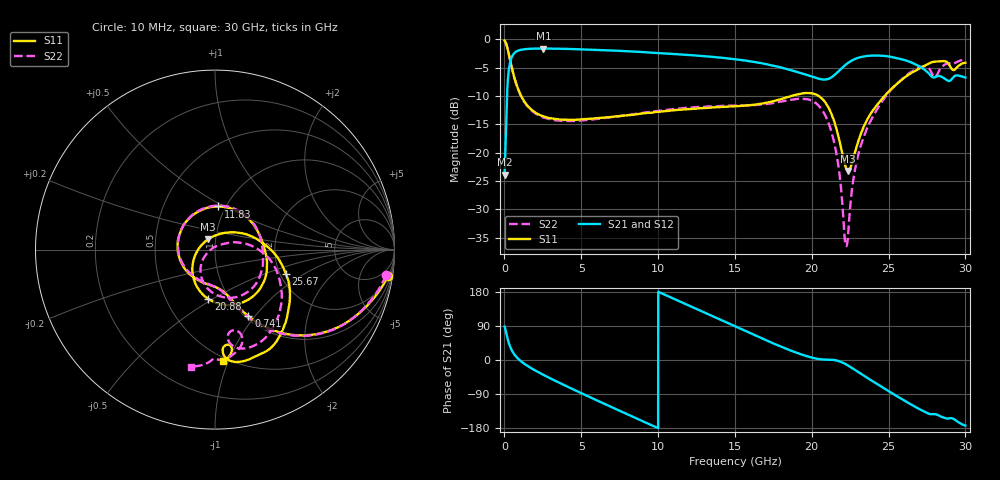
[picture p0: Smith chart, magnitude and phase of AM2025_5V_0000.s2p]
!Keysight Technologies,N5245B,MY58422270,A.16.20.02
!Date: Tuesday, July 14, 2026 00:49:01
!Correction: S11(C  2-Port  )
!S21(C  2-Port  )
!S12(C  2-Port  )
!S22(C  2-Port  )
!S2P File: Measurements: S11, S21, S12, S22:
# Hz S  dB  R 50
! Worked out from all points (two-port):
!   3201 points, 10 MHz to 30 GHz, reference 50 ohm
!   highest |S21| = -1.65 dB at 2.531 GHz (marker M1); lowest = -23.9 dB at 10 MHz (marker M2)
!   |S21| within 3 dB of the highest: 327.9 MHz to 17.47 GHz (17.14 GHz wide, 193 % of centre); 22.14 GHz to 26.91 GHz (4.765 GHz wide, 19.4 % of centre)
!   lowest |S11| = -23.2 dB at 22.37 GHz (marker M3), VSWR 1.15, Z = 46 + j5.25 ohm
!   |S11| at or under -10 dB: 1.086 GHz to 18.69 GHz (17.6 GHz wide, 178 % of centre); 20.45 GHz to 24.74 GHz (4.295 GHz wide, 19 % of centre)
!   |S22| runs from -36.5 to -0.3 dB; largest |S21 - S12| = 0.014
!   S11 on the Smith chart (normalised r, x): 10 MHz: 2, -13; 741 MHz: 1.03, -0.93; 11.83 GHz: 0.92, +0.47; 20.88 GHz: 0.80, -0.48; 25.67 GHz: 2.15, -0.70; 30 GHz: 0.48, -0.96
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1e7  -0.22 -8.7  -23.90 88.2  -23.89 76.5  -0.33 -8.6
3.099e8  -2.95 -41.9  -4.94 41.5  -4.94 41.5  -2.96 -42.3
7.410062e8  -7.65 -63.4  -2.23 9.8  -2.23 9.8  -7.68 -64.3
2.531034e9  -13.62 -89.5  -1.65 -39.2  -1.65 -39.2  -13.79 -91.8
5.014581e9  -14.13 -134.8  -1.78 -87.7  -1.78 -87.8  -14.33 -138.8
7.741797e9  -13.46 168.3  -2.08 -138.5  -2.08 -138.6  -13.48 163.6
1.000979e10  -12.81 121.9  -2.45 180.0  -2.44 179.9  -12.64 116.6
1.182793e10  -12.36 86.0  -2.76 146.9  -2.75 146.9  -12.12 81.2
1.5005e10  -11.82 31.2  -3.53 88.7  -3.53 88.7  -11.69 25.6
1.751666e10  -10.91 -5.0  -4.68 43.4  -4.67 43.3  -11.26 -12.2
2.000958e10  -9.56 -60.8  -6.59 6.3  -6.59 6.2  -10.84 -68.6
2.088117e10  -11.14 -97.8  -7.12 1.2  -7.11 1.1  -13.44 -103.5
2.164966e10  -16.22 -144.1  -5.89 -1.6  -5.89 -1.6  -20.84 -139.5
2.219323e10  -22.42 155.3  -4.53 -10.7  -4.53 -10.7  -36.17 140.3
2.237129e10  -23.23 124.5  -4.16 -14.8  -4.15 -14.8  -34.29 70.2
2.270868e10  -20.97 74.6  -3.61 -23.3  -3.61 -23.4  -24.71 33.5
2.314916e10  -17.04 43.2  -3.18 -34.9  -3.16 -35.0  -19.15 22.0
2.500479e10  -9.25 -6.0  -3.04 -82.4  -3.04 -82.5  -9.44 -14.7
2.567019e10  -7.59 -18.9  -3.42 -98.5  -3.41 -98.6  -7.55 -29.0
2.731964e10  -4.72 -49.1  -5.35 -136.4  -5.34 -136.4  -4.76 -68.7
2.805065e10  -3.95 -64.7  -6.67 -142.9  -6.66 -143.0  -6.69 -76.2
3e10  -4.16 -85.8  -6.76 -173.1  -6.75 -173.3  -3.54 -101.5
